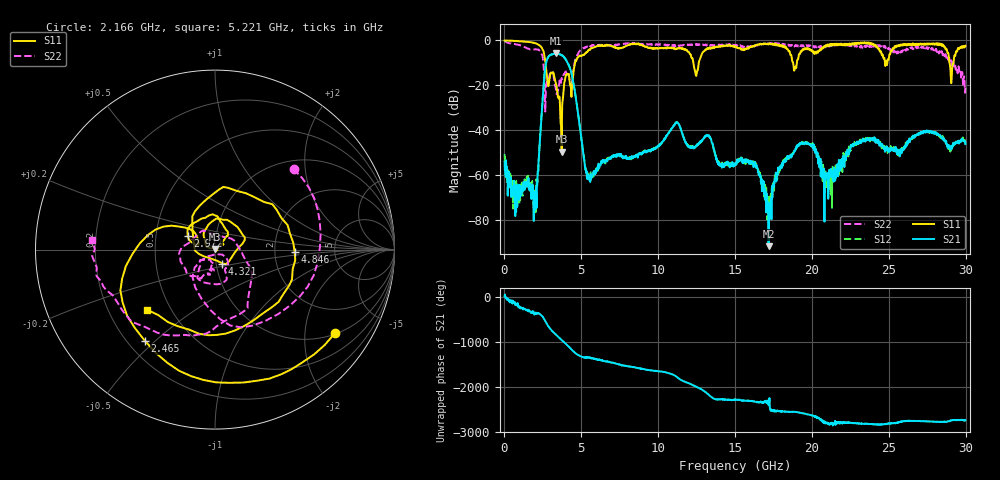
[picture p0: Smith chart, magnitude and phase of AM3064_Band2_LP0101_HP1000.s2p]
# Hz S DB R 50.0
!freq dBS11 angS11 dBS21 angS21 dBS12 angS12 dBS22 angS22
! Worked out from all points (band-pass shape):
!   1600 points, 10 MHz to 29.98 GHz, reference 50 ohm
!   highest |S21| = -5.74 dB at 3.346 GHz (marker M1); lowest = -91.5 dB at 17.18 GHz (marker M2)
!   |S21| within 3 dB of the highest: 2.76 GHz to 4.011 GHz (1.251 GHz wide, 36.9 % of centre)
!   lowest |S11| = -49.5 dB at 3.721 GHz (marker M3), VSWR 1.01, Z = 50.1 + j0.327 ohm
!   |S11| at or under -10 dB: 2.671 GHz to 4.59 GHz (1.919 GHz wide, 52.9 % of centre); 12.29 GHz to 12.64 GHz (354.3 MHz wide, 2.84 % of centre); 28.95 GHz to 29.2 GHz (255.2 MHz wide, 0.878 % of centre)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
!   |S22| runs from -31.7 to -0.3 dB; largest |S21 - S12| = 0.012
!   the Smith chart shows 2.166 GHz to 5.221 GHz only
!   S11 on the Smith chart (normalised r, x): 2.166 GHz: 1.02, -2.84; 2.465 GHz: 0.27, -0.46; 2.972 GHz: 0.73, +0.11; 4.321 GHz: 1.07, -0.17; 4.846 GHz: 2.59, -0.07; 5.221 GHz: 0.37, -0.33
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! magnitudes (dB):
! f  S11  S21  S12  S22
! 10 MHz  0.0  -53.9  -50.5  -0.3
! 703.5 MHz  -0.2  -78.1  -68.6  -1.7
! 2.166 GHz  -1.8  -59.3  -58.0  -4.1
! 2.465 GHz  -3.9  -27.5  -27.6  -6.8
! 2.972 GHz  -15.4  -6.6  -6.5  -14.7
! 3.346 GHz  -19.4  -5.7  -5.8  -22.1
! 3.721 GHz  -49.5  -6.6  -6.5  -16.7
! 4.321 GHz  -21.1  -13.7  -13.6  -21.1
! 4.846 GHz  -7.1  -35.4  -35.3  -5.1
! 5.015 GHz  -7.0  -44.5  -44.2  -4.2
! 5.221 GHz  -5.9  -54.7  -54.5  -3.3
! 10 GHz  -3.5  -47.0  -46.9  -1.9
! 11.24 GHz  -3.8  -36.5  -36.5  -2.6
! 12.46 GHz  -15.7  -47.3  -47.5  -1.8
! 15 GHz  -2.7  -55.4  -54.7  -2.1
! 16.32 GHz  -2.3  -55.0  -54.7  -2.2
! 17.18 GHz  -1.8  -91.5  -72.1  -1.6
! 18.08 GHz  -2.3  -55.6  -55.2  -1.6
! 19.99 GHz  -4.4  -46.6  -47.3  -2.3
! 20.95 GHz  -2.6  -59.5  -59.2  -2.4
! 25 GHz  -8.4  -49.1  -48.2  -3.3
! 29.98 GHz  -2.4  -46.1  -46.3  -20.2
